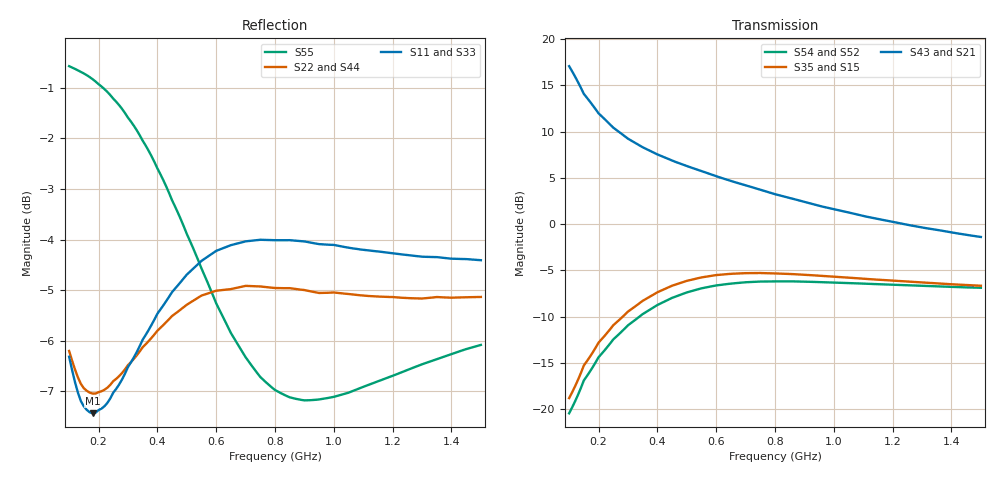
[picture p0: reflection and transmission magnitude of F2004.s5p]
!  POLYFET RF DEVICES
!  S PARAMETERS FOR
!  F2004 (Each Side)
!  VDS=28, IDQ=400mA
! Date: Mon Aug  5 14:04:45 1991
!AWR Design Environment (2053) Wed Feb 04 14:46:15 2004
!freq-unit  param-type  data-format  keyword  impedance-ohms
# MHz  S  MA  R  50
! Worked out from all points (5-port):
!   141 points, 100 MHz to 1.5 GHz, reference 50 ohm
!   strongest paths, dB at 100 MHz, 450 MHz, 800 MHz, 1.15 GHz, 1.5 GHz:
!     S43: 17.1, 6.9, 3.2, 0.5, -1.4
!     S21: 17.1, 6.9, 3.2, 0.5, -1.4
!     S35: -18.8, -6.7, -5.3, -6.0, -6.7
!     S15: -18.8, -6.7, -5.3, -6.0, -6.7
!     S54: -20.5, -8.0, -6.2, -6.5, -6.9
!     S52: -20.5, -8.0, -6.2, -6.5, -6.9
!   lowest |S11| = -7.4 dB at 180 MHz (marker M1), VSWR 2.48, Z = 39.8 - j40.6 ohm
!   |S11| at or under -10 dB: nowhere
